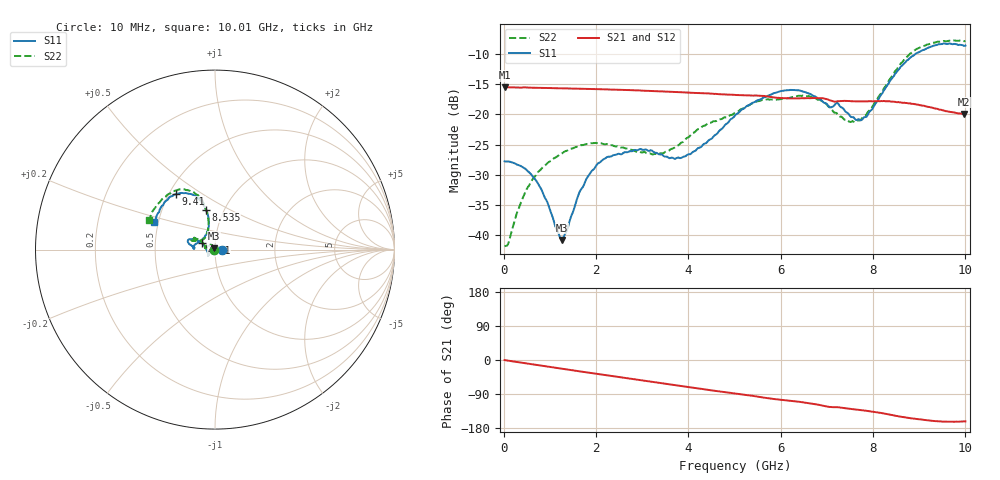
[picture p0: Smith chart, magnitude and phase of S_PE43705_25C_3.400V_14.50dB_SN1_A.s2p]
! Device ID: PE43705
! Serial: 1
! Insertion: A
! Impedance: 50 ohm
! Temp: 25C
! VDD: 3.400V
! Attenuation Step: 14.50dB
#  Hz  S  RI  R  50
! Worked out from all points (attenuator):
!   401 points, 10 MHz to 10.01 GHz, reference 50 ohm
!   highest |S21| = -15.49 dB at 10 MHz (marker M1); lowest = -19.9 dB at 9.985 GHz (marker M2)
!   lowest |S11| = -40.7 dB at 1.26 GHz (marker M3), VSWR 1.02, Z = 49.6 + j0.824 ohm
!   |S11| at or under -10 dB: start of sweep to 8.925 GHz
!   |S22| runs from -41.8 to -7.8 dB; largest |S21 - S12| = 0.0017
!   S11 on the Smith chart (normalised r, x): 10 MHz: 1.09, +0.00; 4.81 GHz: 0.86, +0.06; 8.535 GHz: 0.82, +0.39; 9.41 GHz: 0.54, +0.39; 10.01 GHz: 0.48, +0.17
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1e7  0.0411 0.000113  0.1681 -0.000733  0.1683 -0.000708  -0.00814 0.00053
1.1e8  0.0407 0.00252  0.1675 -0.00627  0.1675 -0.00623  -0.00743 0.00525
4.35e8  0.0342 0.0112  0.1657 -0.024  0.1652 -0.0236  -0.0112 0.0186
6.6e8  0.0255 0.0148  0.1626 -0.0354  0.1626 -0.0353  -0.0174 0.0249
1.26e9  -0.00394 0.0083  0.1512 -0.0647  0.1514 -0.0645  -0.0393 0.0273
1.685e9  -0.0239 -0.00506  0.1401 -0.0835  0.1402 -0.0834  -0.0519 0.0206
2.21e9  -0.0365 -0.0243  0.1232 -0.1039  0.1233 -0.1039  -0.056 0.00984
2.96e9  -0.0386 -0.0345  0.0937 -0.1268  0.0939 -0.1267  -0.048 0.00916
3.36e9  -0.0368 -0.029  0.0766 -0.1352  0.0768 -0.1351  -0.0454 0.0122
3.885e9  -0.044 -0.00737  0.0533 -0.1427  0.0534 -0.1426  -0.0538 0.0249
4.81e9  -0.0744 0.037  0.0122 -0.1459  0.0125 -0.1456  -0.0809 0.0488
5.01e9  -0.0865 0.0467  0.00396 -0.145  0.00405 -0.1452  -0.0888 0.0538
5.985e9  -0.1448 0.0569  -0.0345 -0.1323  -0.0339 -0.1324  -0.1187 0.0613
6.685e9  -0.1414 0.0293  -0.0586 -0.1233  -0.0585 -0.1232  -0.1282 0.0514
7.635e9  -0.0716 0.0549  -0.0839 -0.0971  -0.0836 -0.0972  -0.0548 0.0669
7.885e9  -0.0472 0.0863  -0.0899 -0.0913  -0.09 -0.0922  -0.0427 0.0946
8.36e9  -0.0367 0.1819  -0.104 -0.0759  -0.1035 -0.0759  -0.0411 0.1889
8.535e9  -0.052 0.2231  -0.1071 -0.0671  -0.1066 -0.0683  -0.0549 0.234
8.935e9  -0.1067 0.2999  -0.1103 -0.0503  -0.1102 -0.0498  -0.1234 0.3224
9.41e9  -0.2177 0.3096  -0.1056 -0.0348  -0.1049 -0.0347  -0.2315 0.326
9.985e9  -0.3299 0.1642  -0.0962 -0.0312  -0.0963 -0.0313  -0.3627 0.1764
1.001e10  -0.3374 0.1555  -0.0969 -0.0315  -0.0969 -0.0321  -0.3702 0.1653
